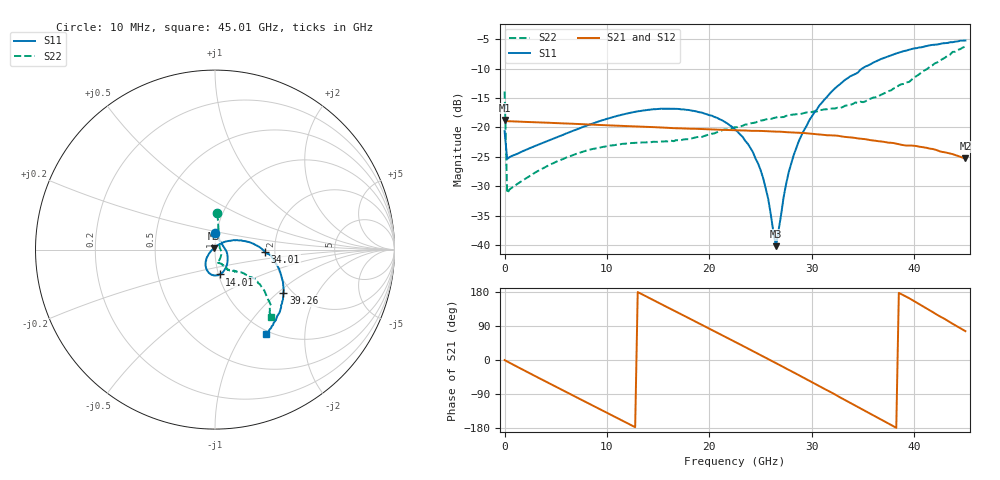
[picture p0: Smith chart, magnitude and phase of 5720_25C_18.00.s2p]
! Device:  ADRF5720
! Description: 0.5dB LSB GaAs MMIC 6-bit Digital Attenuator
! Frequency:  0.000009 -  40 GHz
! Ports:
!	RF1	= Port 1
!	RF2	= Port 2
! Vdd:  3.3 Volt
! Vss:  -3.3 Volt
! Control:  0/3.3 Volt
! State:  18.00 dB attenuation
! Data:  The device was measured using G-S-G Probes on a matrix board.
!  Data was collected using an calibrated 4 port network analyzer.
!  The reference plane for this measurement is at the launchers.
! Note:  Analog Devices supplies this data as a sample of measured data
!  for this product.  Your particular data for this product may vary.
!  Data was taken at 25 degrees C.
!  Analog Devices reserves the right to change this data at anytime.
# GHZ S DB R 45.0
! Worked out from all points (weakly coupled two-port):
!   181 points, 10 MHz to 45.01 GHz, reference 45 ohm
!   highest |S21| = -18.75 dB at 10 MHz (marker M1); lowest = -25.3 dB at 45.01 GHz (marker M2)
!   lowest |S11| = -40.2 dB at 26.51 GHz (marker M3), VSWR 1.02, Z = 44.4 + j0.618 ohm
!   |S11| at or under -10 dB: start of sweep to 34.92 GHz
!   |S22| runs from -31.2 to -6.2 dB; largest |S21 - S12| = 0.00019
!   S11 on the Smith chart (normalised r, x): 10 MHz: 0.98, +0.18; 14.01 GHz: 1.01, -0.29; 34.01 GHz: 1.77, -0.05; 39.26 GHz: 1.81, -1.09; 45.01 GHz: 0.95, -1.28
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0.01  -20.64 90.5  -18.75 -0.2  -18.75 -0.2  -13.90 86.1
0.26  -25.37 8.9  -18.94 -3.9  -18.94 -3.9  -31.19 16.8
3.26  -22.97 -18.0  -19.14 -46.2  -19.14 -46.1  -27.42 -33.9
7.76  -19.86 -47.5  -19.46 -108.4  -19.46 -108.4  -24.07 -66.7
14.01  -17.01 -79.5  -19.92 165.5  -19.92 165.5  -22.53 -78.6
15.26  -16.82 -85.4  -20.00 148.1  -20.00 148.1  -22.42 -77.5
19.26  -17.47 -105.0  -20.28 92.9  -20.28 93.0  -21.62 -68.4
22.76  -20.73 -125.1  -20.50 44.5  -20.50 44.5  -19.96 -61.6
24.01  -23.48 -134.5  -20.58 27.1  -20.58 27.1  -19.32 -60.4
25.01  -27.27 -143.9  -20.60 13.1  -20.60 13.1  -18.84 -59.9
25.76  -32.22 -160.1  -20.66 2.4  -20.66 2.5  -18.56 -59.5
26.51  -40.22 134.5  -20.72 -8.2  -20.72 -8.1  -18.32 -59.6
27.26  -31.85 64.6  -20.77 -19.0  -20.77 -19.0  -18.24 -58.2
27.76  -27.59 49.9  -20.83 -26.0  -20.83 -26.0  -17.95 -58.1
28.76  -22.26 36.3  -20.92 -40.2  -20.92 -40.2  -17.77 -58.0
30.26  -17.46 23.3  -21.11 -62.0  -21.11 -62.0  -17.27 -56.1
32.01  -13.79 10.7  -21.37 -87.0  -21.37 -87.0  -16.79 -53.8
34.01  -11.11 -2.8  -21.74 -116.6  -21.74 -116.6  -16.02 -47.5
37.76  -7.71 -24.2  -22.62 -171.3  -22.62 -171.3  -13.69 -39.5
39.26  -6.92 -32.3  -23.09 166.8  -23.08 166.9  -12.33 -38.7
42.26  -5.89 -46.9  -23.90 119.2  -23.90 119.1  -8.93 -39.7
45.01  -5.20 -59.0  -25.27 76.2  -25.28 76.2  -6.23 -50.3
